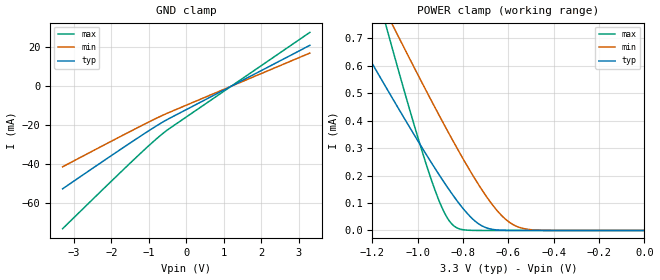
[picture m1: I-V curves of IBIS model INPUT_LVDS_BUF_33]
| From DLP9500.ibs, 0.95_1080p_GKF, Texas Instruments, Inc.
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[Model]   INPUT_LVDS_BUF_33
Model_type  Input
Vinl=0.90
Vinh=1.50
| variable   typ   min   max
C_comp   0.38pF   0.35pF   0.41pF
[Temperature Range]   40   125   -40
| Ambient temperature   25   110   -40
[Voltage range]   3.3   3   3.6
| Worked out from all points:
|   POWER clamp passes 1 mA (typ) near -1.47 V on its own axis
[GND Clamp]
| INPUT_LVDS_BUF_33
|   Voltage   I(typ)   I(min)   I(max)
-3.3V     -52.74mA   -41.43mA   -73.25mA
-1.395V   -27.88mA   -22.26mA   -37.68mA
-600mV    -18.12mA   -14.68mA   -23.91mA
3.3V      21.04mA    17.07mA    27.7mA
[POWER Clamp]
| INPUT_LVDS_BUF_33
|   Voltage   I(typ)   I(min)   I(max)
-3.3V     3.732mA    4.516mA    7.637mA
-1.3V     750.3uA    1.062mA    1.235mA
-1.15V    535.5uA    812.3uA    775.7uA
-1.13V    507.3uA    779.4uA    715.7uA
-1.11V    479.1uA    746.6uA    656.2uA
-930mV    234.1uA    457.4uA    160.7uA
-880mV    170.8uA    380uA      60.86uA
-835mV    117.4uA    312.2uA    13.26uA
-715mV    15.99uA    145.7uA    39.27nA
-635mV    1.157uA    58.78uA    789.5pA
-565mV    86.7nA     15.44uA    104.1pA
-48.03fV  65.94pA    209.5pA    63.77pA
